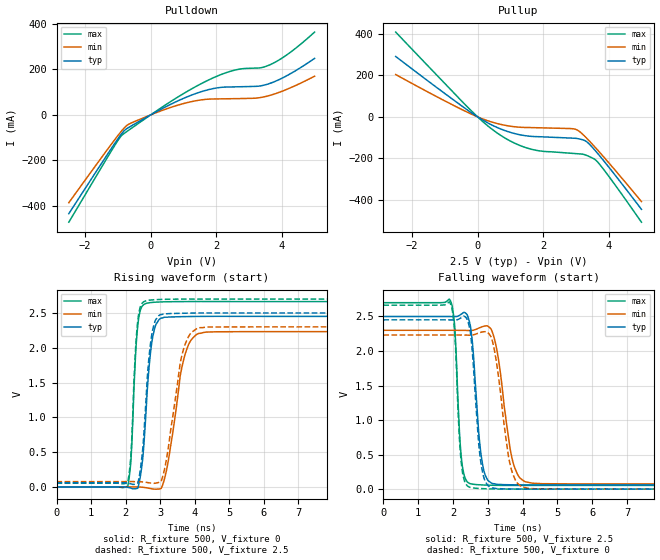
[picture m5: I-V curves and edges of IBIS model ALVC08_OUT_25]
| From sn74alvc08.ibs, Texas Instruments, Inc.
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[Model]   ALVC08_OUT_25
Model_type  Output
Vref =   0
Rref =   500
Cref =   30p
Vmeas =   1.25
| variable   typ   min   max
C_comp   7.89pF   5.59pF   10.52pF
| C_pullup   8.52pF   6.51pF   10.21pF
| C_pulldown   7.27pF   5.59pF   10.52pF
[Temperature Range]   40   100   -40
| Ambient temperature   25   85   -40
[Voltage range]   2.5   2.3   2.7
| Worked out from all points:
|   slope of the pulldown table from 0 to 0.375 V, typ, clamps not added: 12.8 ohm
|   slope of the pullup table from 0 to 0.375 V, typ, clamps not added: 10.9 ohm
|   rising waveform, R_fixture 500, V_fixture 0: 20-80 % time 218ps typ, 401ps min, 148ps max; typ from 0 V to 2.45 V
|   falling waveform, R_fixture 500, V_fixture 2.5: 20-80 % time 218ps typ, 351ps min, 148ps max; typ from 2.5 V to 0.061 V
|   rising waveform, R_fixture 500, V_fixture 2.5: 20-80 % time 213ps typ, 390ps min, 145ps max; typ from 0.061 V to 2.5 V
|   falling waveform, R_fixture 500, V_fixture 0: 20-80 % time 214ps typ, 341ps min, 145ps max; typ from 2.45 V to 0 V
[Pulldown]
| ALVC08_OUT_25
|   Voltage   I(typ)   I(min)   I(max)
-2.5V     -433.6mA   -385.5mA   -471mA
-1.045V   -114.1mA   -98.92mA   -122.1mA
-890mV    -83.15mA   -70.84mA   -91.01mA
-715mV    -59.03mA   -45.2mA    -71.58mA
735mV     55.03mA    38.42mA    69.88mA
1.325V    90.9mA     60.41mA    120.2mA
1.83V     112.9mA    69.33mA    157.4mA
2.53V     122.7mA    70.94mA    195mA
3.37V     127.6mA    76.43mA    206.9mA
3.775V    145.6mA    91.54mA    229.3mA
4.32V     185.2mA    122.2mA    280.8mA
5V        247.8mA    169.5mA    363.1mA
[Pullup]
| ALVC08_OUT_25
|   Voltage   I(typ)   I(min)   I(max)
-2.5V     290.4mA    203.5mA    407.5mA
-235mV    24.72mA    16.51mA    35.93mA
230mV     -22mA      -14.22mA   -32.72mA
660mV     -55.34mA   -34.57mA   -84.31mA
1.155V    -81.27mA   -48.01mA   -128.3mA
1.655V    -93.93mA   -51.65mA   -156.2mA
2.85V     -102mA     -56.39mA   -174.9mA
3.035V    -104mA     -62.79mA   -177.1mA
3.315V    -118.2mA   -100.4mA   -184.6mA
3.645V    -172.4mA   -156.5mA   -214mA
4.1V      -260.8mA   -238.6mA   -306.6mA
5V        -444.6mA   -407.2mA   -506.3mA
[Ramp]
| ALVC08_OUT_25
| variable   typ   min   max
dV/dt_r   1.49/2.26E-10   1.36/4.42E-10   1.60/1.57E-10
dV/dt_f   1.50/2.34E-10   1.37/3.77E-10   1.62/1.60E-10
R_load = 500
[Rising Waveform]
| ALVC08_OUT_25
R_fixture =   500
C_fixture =   0
L_fixture =   0
V_fixture =   0
V_fixture_min = 0
V_fixture_max = 0
|   Time   V(typ)   V(min)   V(max)
0s        34.48pV    4.63nV     26.61pV
2.06ns    -4.977mV   1.254mV    5.363mV
2.15ns    -16.14mV   1.46mV     343.5mV
2.365ns   947.7uV    347uV      2.371V
2.5ns     426.3mV    -4.514mV   2.609V
2.735ns   1.987V     -23.38mV   2.651V
3.13ns    2.439V     123.2mV    2.661V
3.78ns    2.449V     1.991V     2.664V
4.325ns   2.452V     2.225V     2.665V
50ns      2.451V     2.232V     2.664V
[Falling Waveform]
| ALVC08_OUT_25
R_fixture =   500
C_fixture =   0
L_fixture =   0
V_fixture =   2.5
V_fixture_min = 2.3
V_fixture_max = 2.7
|   Time   V(typ)   V(min)   V(max)
0s        2.5V       2.3V       2.7V
1.925ns   2.499V     2.3V       2.728V
2.045ns   2.499V     2.3V       2.383V
2.26ns    2.541V     2.299V     367.5mV
2.615ns   1.743V     2.306V     67.99mV
2.785ns   587.5mV    2.341V     61.71mV
2.975ns   150.7mV    2.366V     57.7mV
3.74ns    61.77mV    361.7mV    53.09mV
4.29ns    60.15mV    84.78mV    53.06mV
50ns      60.54mV    76.61mV    53.33mV
[Rising Waveform]
| ALVC08_OUT_25
R_fixture =   500
C_fixture =   0
L_fixture =   0
V_fixture =   2.5
V_fixture_min = 2.3
V_fixture_max = 2.7
|   Time   V(typ)   V(min)   V(max)
0s        60.54mV    76.61mV    53.33mV
2.06ns    55.47mV    77.74mV    63.9mV
2.15ns    45.44mV    77.85mV    420.2mV
2.36ns    65.31mV    76.65mV    2.416V
2.5ns     563.7mV    71.86mV    2.65V
2.715ns   2.032V     57.45mV    2.686V
3.055ns   2.479V     116.9mV    2.696V
3.645ns   2.496V     1.921V     2.7V
4.16ns    2.5V       2.29V      2.7V
50ns      2.5V       2.3V       2.7V
[Falling Waveform]
| ALVC08_OUT_25
R_fixture =   500
C_fixture =   0
L_fixture =   0
V_fixture =   0
V_fixture_min = 0
V_fixture_max = 0
|   Time   V(typ)   V(min)   V(max)
0s        2.451V     2.232V     2.664V
1.92ns    2.451V     2.232V     2.691V
2.045ns   2.451V     2.232V     2.311V
2.26ns    2.49V      2.231V     285.6mV
2.61ns    1.6V       2.238V     14.4mV
2.92ns    120.1mV    2.28V      4.947mV
3.19ns    13.1mV     2.014V     1.71mV
3.68ns    1.568mV    280.2mV    -143.1uV
4.18ns    -288.3uV   10.12mV    -289.5uV
50ns      35.93pV    4.629nV    26.96pV
